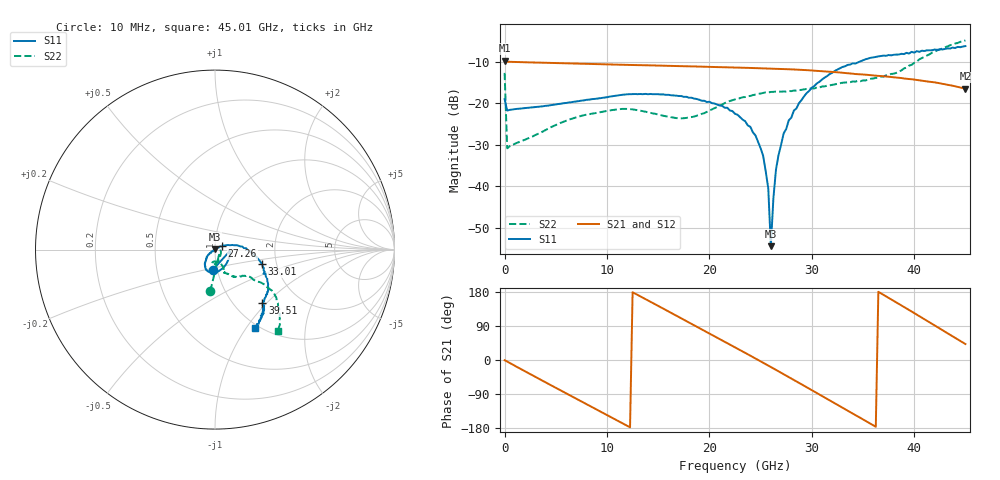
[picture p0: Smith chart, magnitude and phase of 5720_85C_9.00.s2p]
! Device:  ADRF5720
! Description: 0.5dB LSB GaAs MMIC 6-bit Digital Attenuator
! Frequency:  0.000009 -  40 GHz
! Ports:
!	RF1	= Port 1
!	RF2	= Port 2
! Vdd:  3.3 Volt
! Vss:  -3.3 Volt
! Control:  0/3.3 Volt
! State:  9.00 dB attenuation
! Data:  The device was measured using G-S-G Probes on a matrix board.
!  Data was collected using an calibrated 4 port network analyzer.
!  The reference plane for this measurement is at the launchers.
! Note:  Analog Devices supplies this data as a sample of measured data
!  for this product.  Your particular data for this product may vary.
!  Data was taken at 85 degrees C.
!  Analog Devices reserves the right to change this data at anytime.
# GHZ S DB R 45.0
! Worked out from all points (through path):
!   181 points, 10 MHz to 45.01 GHz, reference 45 ohm
!   highest |S21| = -9.67 dB at 10 MHz (marker M1); lowest = -16.5 dB at 45.01 GHz (marker M2)
!   group delay of S21, straight-line fit = 41.5 ps
!   lowest |S11| = -54.5 dB at 26.01 GHz (marker M3), VSWR 1.00, Z = 45 + j0.163 ohm
!   |S11| at or under -10 dB: start of sweep to 34.63 GHz
!   |S22| runs from -30.9 to -4.8 dB; largest |S21 - S12| = 0.0015
!   S11 on the Smith chart (normalised r, x): 10 MHz: 0.95, -0.22; 27.26 GHz: 1.08, +0.04; 33.01 GHz: 1.68, -0.29; 39.51 GHz: 1.34, -0.95; 45.01 GHz: 0.96, -1.10
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0.01  -18.98 -95.9  -9.67 -0.6  -9.66 -0.6  -12.66 -96.5
0.26  -21.75 -7.2  -9.96 -4.0  -9.95 -4.0  -30.87 -16.4
4.26  -20.56 -38.0  -10.23 -62.6  -10.21 -62.5  -26.15 -56.4
7.76  -19.30 -62.2  -10.45 -113.0  -10.43 -113.0  -22.88 -79.3
11.51  -17.94 -85.4  -10.69 -166.8  -10.68 -166.7  -21.35 -96.7
15.26  -17.86 -105.5  -10.90 139.1  -10.89 139.3  -22.85 -101.0
19.01  -19.13 -119.7  -11.13 84.8  -11.11 85.0  -22.84 -74.2
22.76  -22.77 -131.6  -11.38 29.9  -11.36 30.1  -18.90 -65.6
24.01  -25.68 -140.8  -11.46 11.4  -11.45 11.6  -18.21 -67.3
25.26  -32.70 -151.9  -11.55 -7.2  -11.53 -7.0  -17.49 -68.6
25.76  -40.55 -158.4  -11.58 -14.7  -11.57 -14.5  -17.39 -68.8
26.01  -54.51 74.4  -11.60 -18.5  -11.59 -18.2  -17.26 -68.7
26.26  -42.91 41.0  -11.62 -22.2  -11.60 -22.0  -17.24 -68.4
26.51  -36.07 37.2  -11.64 -26.1  -11.63 -25.8  -17.16 -68.1
27.26  -27.27 24.4  -11.72 -37.5  -11.70 -37.2  -17.14 -67.8
28.26  -21.75 18.1  -11.83 -52.7  -11.82 -52.4  -16.93 -66.6
30.26  -15.83 2.7  -12.12 -83.4  -12.10 -83.1  -16.41 -62.5
33.01  -11.22 -17.2  -12.63 -126.0  -12.61 -125.7  -15.03 -57.1
37.76  -8.42 -41.4  -13.66 160.0  -13.64 160.4  -12.91 -40.8
39.51  -7.99 -48.4  -14.14 132.0  -14.12 132.4  -10.90 -37.6
42.01  -7.00 -52.5  -14.94 91.4  -14.92 91.8  -7.55 -37.3
45.01  -6.19 -62.9  -16.47 42.1  -16.45 42.5  -4.82 -52.0
